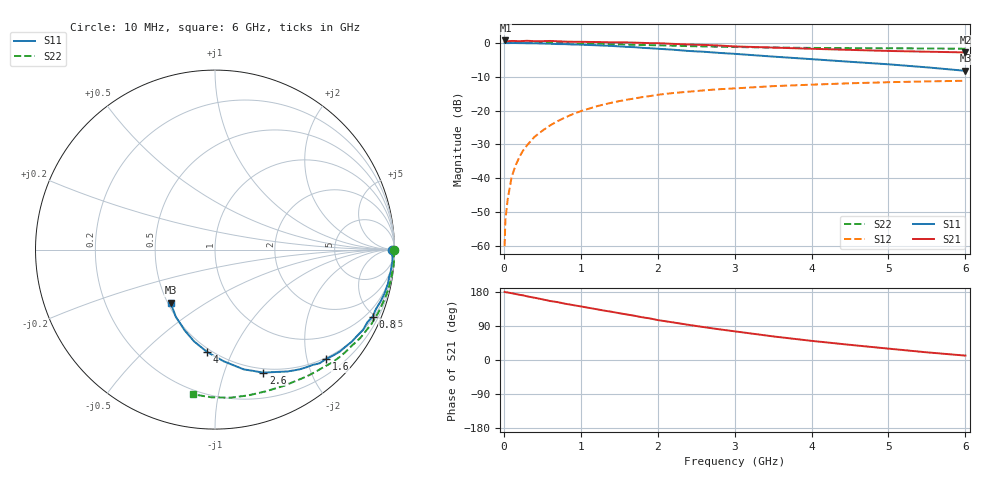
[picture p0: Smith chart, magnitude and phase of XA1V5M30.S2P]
! SIEMENS Discrete & RF Semiconductors
! BFY180
! Si NPN RF Bipolar Junction Transistor in MICRO-X
! VCE = 1.5 V  IC = 0.3 mA
! Common Emitter S-Parameters:  May  1997
# GHz  S  MA  R  50
!  f  S11  S21  S12  S22
! GHz  MAG  ANG  MAG  ANG  MAG  ANG  MAG  ANG
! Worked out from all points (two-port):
!   36 points, 10 MHz to 6 GHz, reference 50 ohm
!   highest |S21| = 0.68 dB at 20 MHz (marker M1); lowest = -2.9 dB at 6 GHz (marker M2)
!   |S21| within 3 dB of the highest: start of sweep to 4.85 GHz
!   lowest |S11| = -8.3 dB at 6 GHz (marker M3), VSWR 2.26, Z = 25.9 - j18 ohm
!   |S11| at or under -10 dB: nowhere
!   |S22| runs from -1.8 to 0.0 dB; largest |S21 - S12| = 1.1
!   S11 on the Smith chart (normalised r, x): 10 MHz: open; 800 MHz: 0.58, -4.85; 1.6 GHz: 0.47, -2.36; 2.6 GHz: 0.46, -1.36; 4 GHz: 0.48, -0.81; 6 GHz: 0.52, -0.36
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0.01  0.9882 -0.2  1.049 179.8  0.001 100.7  0.9986 -0.2
0.02  0.9896 -0.4  1.081 179.0  0.0024 88.9  0.9999 -0.5
0.05  0.9874 -1.4  1.053 178.2  0.0049 88.3  0.9999 -1.0
0.1  0.9903 -2.9  1.063 176.3  0.0103 89.7  0.9968 -2.2
0.15  0.9901 -4.5  1.061 174.3  0.0153 87.9  0.9993 -3.2
0.25  0.9869 -7.3  1.06 170.6  0.0258 85.0  0.999 -5.4
0.3  0.982 -8.6  1.07 168.1  0.0306 83.0  0.996 -6.4
0.4  0.982 -11.3  1.055 164.3  0.0411 80.9  0.9952 -8.5
0.6  0.967 -17.3  1.063 155.7  0.0603 76.1  0.9903 -12.8
0.8  0.9542 -23.0  1.039 148.4  0.0793 70.9  0.9826 -17.1
1.1  0.9271 -31.0  1.028 137.8  0.1061 64.1  0.969 -23.2
1.4  0.8974 -39.4  1.014 127.3  0.1304 57.1  0.9521 -29.4
1.6  0.8685 -44.6  1.011 120.1  0.1445 53.2  0.9396 -33.2
2  0.8161 -54.9  0.986 105.4  0.1709 45.5  0.9184 -40.3
2.2  0.7897 -59.3  0.963 99.2  0.1813 41.5  0.9069 -43.9
2.6  0.7365 -68.6  0.93 86.8  0.1984 35.1  0.8827 -50.2
2.8  0.7084 -72.5  0.91 81.0  0.2065 32.0  0.8741 -53.3
3.5  0.625 -85.4  0.849 62.3  0.2291 22.6  0.8504 -63.2
4  0.5729 -94.3  0.815 50.5  0.241 16.4  0.8389 -70.2
4.5  0.5241 -102.9  0.785 40.0  0.2524 10.7  0.8331 -77.2
5.5  0.4337 -120.2  0.738 20.2  0.2691 0.0  0.8231 -91.4
6  0.3856 -130.0  0.72 11.6  0.275 -5.5  0.8158 -98.5
